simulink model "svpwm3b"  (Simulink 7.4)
settings: Solver=ode45  StartTime=0  StopTime=.02  MaxStep=1e-6  RelTol=1e-2
InitFcn:
  | clc;fout=50;fsw=10000;disp(' Output frequency Switching frequency  [Hz] :  ');
  | disp('         fout       fsw');disp([fout   fsw])
libraries: simulink x2

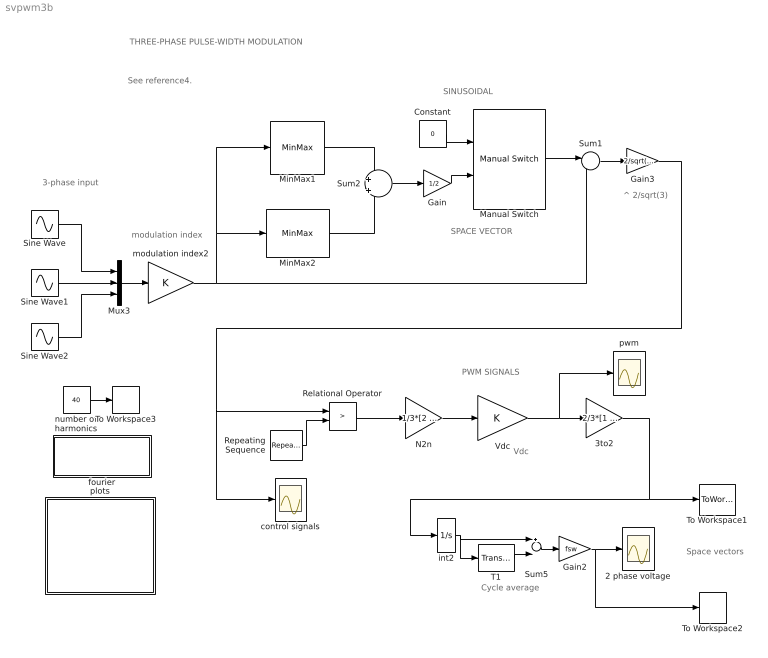
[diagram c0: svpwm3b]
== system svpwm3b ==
  note: SINUSOIDAL
  note: modulation index
  note: THREE-PHASE PULSE-WIDTH MODULATION
  note: 3-phase input
  note: See reference4.
  note: SPACE VECTOR
  note: Cycle average
  note: PWM SIGNALS
  note: ^ 2/sqrt(3)
  note: Vdc
  note: Space vectors
  2 phase voltage : Scope
  3to2 : Gain  Gain=2/3*[1 -0.5 -0.5;0 sqrt(3)/2 -sqrt(3)/2]  Multiplication=Matrix(K*u)  ParameterDataType=sfix(16)  ParameterScaling=2^0  OutDataType=sfix(16)  OutScaling=2^0
  Constant : Constant  Value=0  OutDataType=sfix(16)  OutScaling=2^0
  Gain : Gain  Gain=1/2  ParameterDataType=sfix(16)  ParameterScaling=2^0  OutDataType=sfix(16)  OutScaling=2^0
  Gain2 : Gain  Gain=fsw  ParameterDataType=sfix(16)  ParameterScaling=2^0  OutDataType=sfix(16)  OutScaling=2^0
  Gain3 : Gain  Gain=2/sqrt(3)  ParameterDataType=sfix(16)  ParameterScaling=2^0  OutDataType=sfix(16)  OutScaling=2^0
  Manual Switch : simulink/Signal Routing/Manual Switch  SystemSampleTime=-1  sw=0  action=0  varsize=off
  MinMax1 : MinMax
  MinMax2 : MinMax  Function=max
  Mux3 : Mux  Inputs=3
  N2n : Gain  Gain=1/3*[2 -1 -1;-1 2 -1;-1 -1 2]  Multiplication=Matrix(K*u)  ParameterDataType=sfix(16)  ParameterScaling=2^0  OutDataType=sfix(16)  OutScaling=2^0
  Relational Operator : RelationalOperator  Operator=>
  Repeating Sequence : simulink/Sources/Repeating Sequence  SystemSampleTime=-1  rep_seq_t="[0  0.5/fsw 1/fsw]"  rep_seq_y=[1 -1 1]
  Sine Wave : Sin  Amplitude=1  Bias=0  Frequency=2*pi*fout  Phase=pi/2  Samples=10  SampleTime=0
  Sine Wave1 : Sin  Amplitude=1  Bias=0  Frequency=2*pi*fout  Phase=pi/2 -2*pi/3  Samples=10  SampleTime=0
  Sine Wave2 : Sin  Amplitude=1  Bias=0  Frequency=2*pi*fout  Phase=pi/2+2*pi/3  Samples=10  SampleTime=0
  Sum1 : Sum  Inputs=|-+  OutDataType=sfix(16)  OutScaling=2^0
  Sum2 : Sum  Inputs=+|+  OutDataType=sfix(16)  OutScaling=2^0
  Sum5 : Sum  Inputs=+-  OutDataType=sfix(16)  OutScaling=2^0
  T1 : TransportDelay  DelayTime=1/fsw
  To Workspace1 : ToWorkspace  VariableName=abpwm  SampleTime=-1  SaveFormat=Array
  To Workspace2 : ToWorkspace  VariableName=ab  SampleTime=-1  SaveFormat=Array
  To Workspace3 : ToWorkspace  VariableName=h  SampleTime=-1  SaveFormat=Array
  Vdc : Gain  ParameterDataType=sfix(16)  ParameterScaling=2^0  OutDataType=sfix(16)  OutScaling=2^0
  control signals : Scope
  fourier : Subsystem
  int2 : Integrator
  modulation index2 : Gain  ParameterDataType=sfix(16)  ParameterScaling=2^0  OutDataType=sfix(16)  OutScaling=2^0
  number of harmonics : Constant  Value=40  OutDataType=sfix(16)  OutScaling=2^0
  plots : Subsystem
  pwm : Scope
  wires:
  Sine Wave/1 -> Mux3/1
  Sine Wave1/1 -> Mux3/2
  Sine Wave2/1 -> Mux3/3
  Mux3/1 -> modulation index2/1
  Sum1/1 -> Gain3/1
  modulation index2/1 -> MinMax2/1, MinMax1/1, Sum1/2
  Sum2/1 -> Gain/1
  MinMax1/1 -> Sum2/1
  MinMax2/1 -> Sum2/2
  Manual Switch/1 -> Sum1/1
  Gain/1 -> Manual Switch/2
  Constant/1 -> Manual Switch/1
  Repeating Sequence/1 -> Relational Operator/2
  T1/1 -> Sum5/2
  int2/1 -> Sum5/1, T1/1
  Sum5/1 -> Gain2/1
  Gain2/1 -> 2 phase voltage/1, To Workspace2/1
  Vdc/1 -> 3to2/1, pwm/1
  Gain3/1 -> control signals/1, Relational Operator/1
  3to2/1 -> int2/1, To Workspace1/1
  number of harmonics/1 -> To Workspace3/1
  Relational Operator/1 -> N2n/1
  N2n/1 -> Vdc/1

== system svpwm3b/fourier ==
  note: To obtain the Fourier decomposition of a periodic signal: a) run a simulation for one period duration b) Specify the fundamental frequency c) Specify the number of harmonics

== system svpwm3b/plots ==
